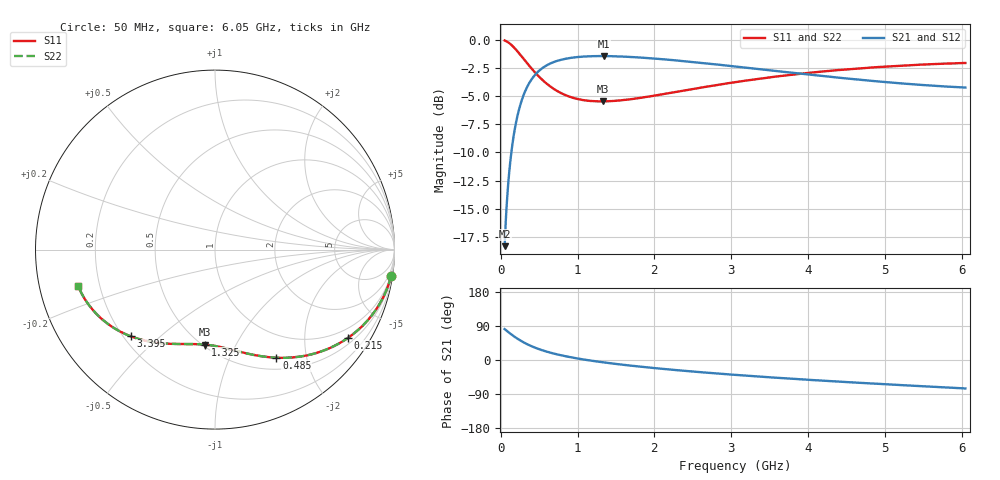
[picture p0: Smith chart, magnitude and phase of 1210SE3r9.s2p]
! AVX Thin Film Operation		Date: August 2001
! Description: Accu-P® Series, Thin Film, SMD, RF Capacitor
! Part Number: 12101J3R9ABT
! 50 MHz  -  6.05 GHz
! Serial Measurements
# mhz S db R 50
!	S11		S21		S12		S22
!	dB	Phase	dB	Phase	dB	Phase	dB	Phase
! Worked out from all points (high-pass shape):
!   401 points, 50 MHz to 6.05 GHz, reference 50 ohm
!   highest |S21| = -1.45 dB at 1.34 GHz (marker M1); lowest = -18.3 dB at 50 MHz (marker M2)
!   |S21| within 3 dB of the highest: 325.4 MHz to end of sweep
!   lowest |S11| = -5.5 dB at 1.325 GHz (marker M3), VSWR 3.28, Z = 25.7 - j38 ohm
!   |S11| at or under -10 dB: nowhere
!   |S22| runs from -5.5 to -0.1 dB; largest |S21 - S12| = 0
!   S11 on the Smith chart (normalised r, x): 50 MHz: 1, -14; 215 MHz: 0.68, -3.20; 485 MHz: 0.65, -1.51; 1.325 GHz: 0.51, -0.76; 3.395 GHz: 0.23, -0.40; 6.05 GHz: 0.12, -0.13
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50  -0.06 -8.4  -18.33 81.6  -18.33 81.6  -0.06 -8.4
125  -0.38 -20.5  -10.76 69.5  -10.76 69.5  -0.38 -20.5
170  -0.67 -27.2  -8.44 62.7  -8.44 62.7  -0.67 -27.2
215  -1.01 -33.4  -6.83 56.5  -6.83 56.5  -1.01 -33.4
275  -1.51 -40.9  -5.33 49.1  -5.33 49.1  -1.51 -40.9
335  -2.02 -47.4  -4.31 42.6  -4.31 42.6  -2.02 -47.4
410  -2.63 -54.4  -3.43 35.6  -3.43 35.6  -2.63 -54.4
485  -3.19 -60.4  -2.84 29.6  -2.84 29.6  -3.19 -60.4
590  -3.86 -67.4  -2.30 22.6  -2.30 22.6  -3.86 -67.4
725  -4.51 -74.7  -1.90 15.3  -1.90 15.3  -4.51 -74.7
875  -5.01 -81.3  -1.65 8.7  -1.65 8.7  -5.01 -81.3
1055  -5.34 -87.9  -1.50 2.1  -1.50 2.1  -5.34 -87.9
1325  -5.48 -95.9  -1.45 -5.9  -1.45 -5.9  -5.48 -95.9
1340  -5.48 -96.3  -1.45 -6.3  -1.45 -6.3  -5.48 -96.3
1685  -5.29 -104.7  -1.53 -14.7  -1.53 -14.7  -5.29 -104.7
2060  -4.90 -112.5  -1.70 -22.5  -1.70 -22.5  -4.90 -112.5
2540  -4.33 -121.1  -2.00 -31.1  -2.00 -31.1  -4.33 -121.1
3050  -3.77 -129.2  -2.37 -39.2  -2.37 -39.2  -3.77 -129.2
3395  -3.44 -134.1  -2.63 -44.2  -2.63 -44.2  -3.44 -134.1
4055  -2.91 -142.8  -3.12 -52.8  -3.12 -52.8  -2.91 -142.8
5060  -2.36 -154.5  -3.79 -64.6  -3.79 -64.6  -2.36 -154.5
6050  -2.06 -165.0  -4.25 -75.1  -4.25 -75.1  -2.06 -165.0
